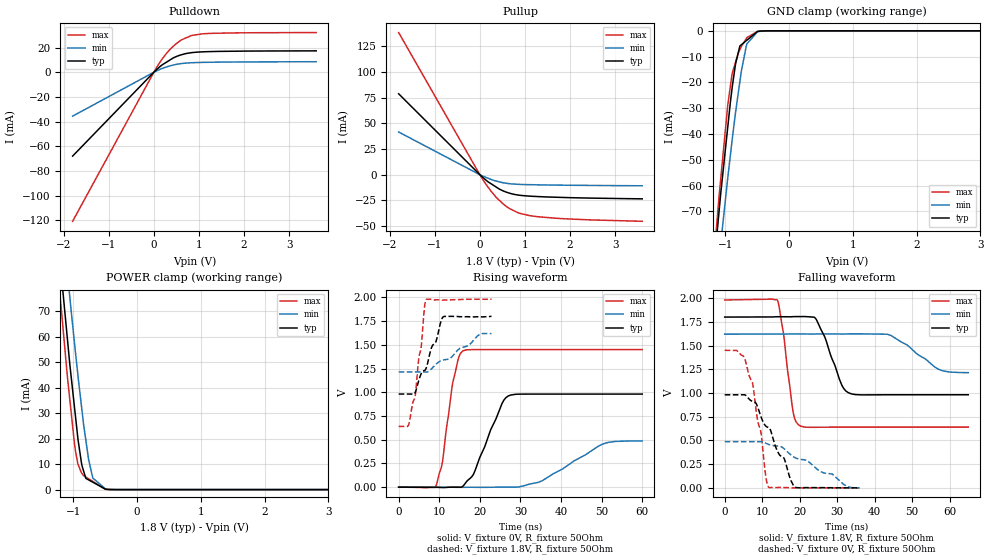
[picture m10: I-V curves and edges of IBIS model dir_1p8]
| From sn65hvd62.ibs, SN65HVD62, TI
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|   dir_1p8 Model
[Model]   dir_1p8
Model_type   3-state
Polarity   Non-Inverting
Vmeas = 0.9
Vref = 0.9
Cref = 2pF
Rref = 50
|   typ   min   max
|   (nom PVT)   (fast PVT)   (slow PVT)
 C_comp   2.130e-12   2.001e-12   2.343e-12
|ON state : BUFFER OUTPUT TURNED HIGH
|C_comp   2.130e-12   2.001e-12   2.343e-12
|OFF state: BUFFER IN HIGH IMPEDANCE
|C_comp   1.738e-12   1.711e-12   1.756e-12
| Where nom  PVT is Nominal Process, 1.8V, 27C
|   Fast PVT is Strong Process,  1.98V, -40C
|   Slow PVT is Weak Process,   1.62V, 125C
[Voltage Range]   1.8   1.62   1.98
|Ambient Temperature   25   85   -40
|Junction Temperature
[Temperature Range]   27   125   -40
[Pullup Reference]   1.8   1.62   1.98
[Pulldown Reference]   0   0   0
[Power Clamp Reference]   1.8   1.62   1.98
[GND Clamp Reference]   0   0   0
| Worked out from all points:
|   slope of the pulldown table from 0 to 0.27 V, typ, clamps not added: 34 ohm
|   slope of the pullup table from 0 to 0.27 V, typ, clamps not added: 28.7 ohm
|   GND clamp passes 1 mA (typ) near -0.53 V on its own axis
|   POWER clamp passes 1 mA (typ) near -0.55 V on its own axis
|   falling waveform, V_fixture 1.8V, R_fixture 50Ohm: 20-80 % time 4.5ns typ, 8.33ns min, 2.54ns max; typ from 1.8 V to 0.981 V
|   rising waveform, V_fixture 0V, R_fixture 50Ohm: 20-80 % time 5.57ns typ, 11.2ns min, 2.79ns max; typ from 0 V to 0.981 V
|   rising waveform, V_fixture 1.8V, R_fixture 50Ohm: 20-80 % time 4.69ns typ, 9.05ns min, 2.37ns max; typ from 0.981 V to 1.8 V
|   falling waveform, V_fixture 0V, R_fixture 50Ohm: 20-80 % time 7.36ns typ, 13.6ns min, 3.69ns max; typ from 0.981 V to 0 V
[Pulldown]
|   Voltage   I(typ)   I(min)   I(max)
-1.8V     -67.98mA   -35.58mA   -120.9mA
11.88mV   416uA      214.2uA    777.5uA
156.4mV   5.193mA    2.663mA    9.304mA
269.3mV   7.928mA    4.204mA    14.83mA
499mV     12.75mA    6.41mA     23.29mA
623.7mV   14.31mA    7.127mA    26.46mA
823.7mV   15.83mA    7.699mA    29.65mA
1.069V    16.56mA    8.011mA    31.15mA
1.869V    17.11mA    8.35mA     31.97mA
3.6V      17.36mA    8.563mA    32.21mA
[GND Clamp]
|   Voltage   I(typ)   I(min)   I(max)
-1.8V     -270.6mA   -265.6mA   -290.4mA
-1.168V   -88.77mA   -105mA     -85.35mA
-1.099V   -70.45mA   -89mA      -64.65mA
-1.071V   -63.06mA   -82.53mA   -57.4mA
-958.3mV  -36.73mA   -56.48mA   -28.26mA
-891mV    -21.84mA   -42.08mA   -16.46mA
-837mV    -12.64mA   -31.33mA   -12mA
-770.4mV  -5.858mA   -19.57mA   -7.292mA
-748.4mV  -5.411mA   -15.69mA   -6.075mA
-672.3mV  -3.86mA    -6.122mA   -3.093mA
-495mV    -249.2uA   -377.1uA   -244.2uA
3.6V      0A         0A         0A
[Pullup]
|   Voltage   I(typ)   I(min)   I(max)
-1.8V     78.8mA     41.59mA    138.4mA
9.9mV     -396.9uA   -212.1uA   -728.9uA
132.7mV   -5.164mA   -2.531mA   -9.159mA
348.5mV   -11.63mA   -5.981mA   -21.31mA
601.9mV   -17.2mA    -8.411mA   -31.38mA
871.2mV   -19.95mA   -9.414mA   -37.47mA
1.277V    -21.26mA   -9.842mA   -40.87mA
2.376V    -22.71mA   -10.42mA   -43.87mA
3.6V      -23.51mA   -10.79mA   -45.37mA
[POWER Clamp]
|   Voltage   I(typ)   I(min)   I(max)
-1.8V     258.3mA    274.1mA    254.6mA
-1.238V   97.88mA    123.8mA    85.15mA
-1.131V   69.54mA    94.98mA    55.24mA
-1.053V   49.06mA    75.32mA    35.26mA
-982.1mV  32.77mA    57.96mA    18.46mA
-928.6mV  20.48mA    45.39mA    10.24mA
-862.2mV  9.373mA    30.92mA    6.288mA
-802.8mV  4.428mA    19.48mA    4.957mA
-759.8mV  3.833mA    11.93mA    4.282mA
-693.4mV  2.916mA    4.575mA    3.239mA
-495mV    176.7uA    269.3uA    126.9uA
3.6V      0A         0A         0A
[Ramp]
R_load = 50
|   typ   min   max
dV/dt_r   0.588465/5.56017e-09   0.292116/1.11649e-08   0.869682/2.78212e-09
dV/dt_f   0.491337/4.5101e-09   0.243332/8.2918e-09   0.804055/2.53979e-09
[Falling Waveform]
V_fixture = 1.8V
V_fixture_min = 1.62V
V_fixture_max = 1.98V
R_fixture = 50Ohm
|   Time   V(typ)   V(min)   V(max)
0s        1.8V       1.62V      1.98V
14.1ns    1.804V     1.621V     1.976V
15.73ns   1.803V     1.62V      1.617V
18.27ns   1.805V     1.622V     798.1mV
20.3ns    1.805V     1.622V     650.2mV
24.26ns   1.785V     1.622V     638.5mV
32.94ns   1.004V     1.623V     639.9mV
43.39ns   981.1mV    1.619V     639.9mV
57.02ns   981.1mV    1.25V      639.9mV
64.98ns   981.1mV    1.214V     639.9mV
[Rising Waveform]
V_fixture = 0V
V_fixture_min = 0V
V_fixture_max = 0V
R_fixture = 50Ohm
|   Time   V(typ)   V(min)   V(max)
0s        3.488nV    33.09nV    2.351nV
9.184ns   -1.936mV   -1.017mV   10.65mV
10.77ns   -4.094mV   -947.3uV   259.9mV
13.38ns   -91.31uV   -1.04mV    1.112V
15.79ns   8.843mV    -1.558mV   1.434V
18.43ns   136.2mV    -1.292mV   1.449V
26.93ns   959.1mV    8.492uV    1.449V
35.32ns   980.8mV    66.31mV    1.449V
50.26ns   980.8mV    454.2mV    1.449V
60ns      980.8mV    486.9mV    1.449V
[Rising Waveform]
V_fixture = 1.8V
V_fixture_min = 1.62V
V_fixture_max = 1.98V
R_fixture = 50Ohm
|   Time   V(typ)   V(min)   V(max)
0s        981.1mV    1.214V     639.9mV
2.352ns   981.1mV    1.214V     645.6mV
3.984ns   989.6mV    1.214V     944mV
4.928ns   1.12V      1.214V     1.348V
5.584ns   1.199V     1.214V     1.492V
6.376ns   1.228V     1.214V     1.901V
6.744ns   1.251V     1.213V     1.976V
10.86ns   1.791V     1.339V     1.97V
20.04ns   1.796V     1.611V     1.98V
22.88ns   1.8V       1.618V     1.98V
[Falling Waveform]
V_fixture = 0V
V_fixture_min = 0V
V_fixture_max = 0V
R_fixture = 50Ohm
|   Time   V(typ)   V(min)   V(max)
0s        980.8mV    486.9mV    1.449V
5ns       980.9mV    486.9mV    1.388V
7.344ns   912.2mV    486.9mV    1.119V
8.728ns   859.8mV    486.8mV    724.4mV
9.712ns   746.9mV    487.2mV    573mV
10.8ns    658.6mV    474mV      167.4mV
11.62ns   637.6mV    459.6mV    12mV
19ns      3.36mV     314.3mV    169.9uV
32.74ns   38uV       14.11mV    13.14nV
35.98ns   4.042nV    117.9nV    2.353nV
